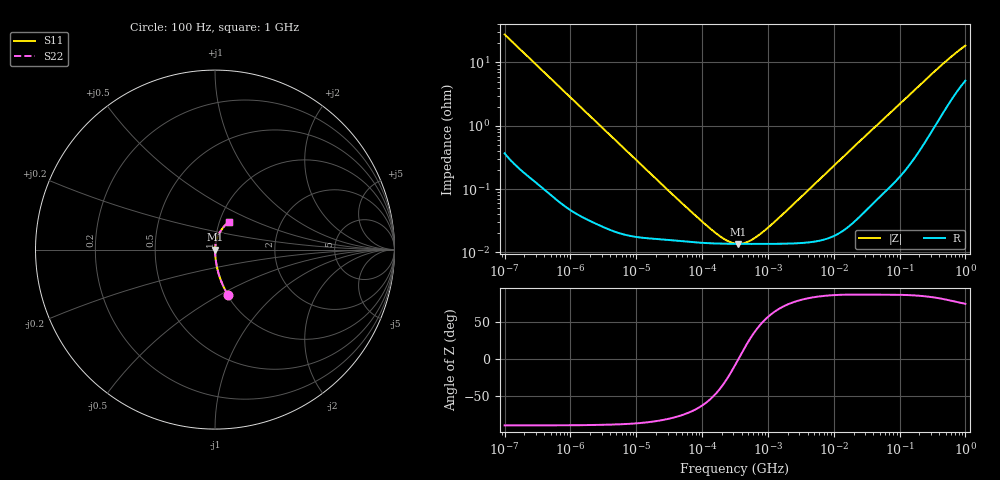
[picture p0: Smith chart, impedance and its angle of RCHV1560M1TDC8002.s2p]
! RCHV1560M1TDC8002  S-PARAMETER MODEL  (AEC-Q200 qualified)
! Model Generated by ELNA Corporation (http://www.ty-top.com)
! Version 1.0
! ELNA Control No. 240229
! Copyright (c) 2024 ELNA CO.,LTD. All Rights Reserved.
! Products Name : CONDUCTIVE POLYMER HYBRID ALUMINUM ELECTROLYTIC CAPACITORS
! Characteristics :
!  Capacitance  :  56uF  ,  Rated voltage  :  25V
!  Operating Temp. Range  :  -55 to +105 degC  ,  Endurance  :  5000hr at 105 degC
!  Dimension D  :  6.3mm  ,  Dimension L  :  5.8mm
! Frequency Range : 100Hz - 1GHz
! External Node Assignments :
!  1  o---| |---o  2
# MHz S RI R 50
!Freq[MHz].  S11 Real  S11 Imag  S21 Real  S21 Imag  S12 Real  S12 Imag  S22 Real  S22 Imag
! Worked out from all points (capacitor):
!   401 points, 100 Hz to 1 GHz, reference 50 ohm
!   read as one part in series: C = 57.5 uF near 108 Hz
!   lowest |Z| = 13.6 mohm at 356.9 kHz (marker M1)
!   series resonance near 357.6 kHz, so ESL is about 3.4 nH
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0.0001  0.074 -0.2553  0.926 0.2553  0.926 0.2553  0.074 -0.2553
0.000113  0.0594 -0.23  0.9406 0.23  0.9406 0.23  0.0594 -0.23
0.000183  0.0242 -0.1476  0.9758 0.1476  0.9758 0.1476  0.0242 -0.1476
0.000309  0.00924 -0.0891  0.9908 0.0891  0.9908 0.0891  0.00924 -0.0891
0.000613  0.00275 -0.0455  0.9972 0.0455  0.9972 0.0455  0.00275 -0.0455
0.001488  0.000722 -0.0189  0.9993 0.0189  0.9993 0.0189  0.000722 -0.0189
0.022131  0.000163 -0.00129  0.9998 0.00129  0.9998 0.00129  0.000163 -0.00129
0.074131  0.000145 -0.00038  0.9999 0.00038  0.9999 0.00038  0.000145 -0.00038
0.147062  0.000139 -0.000168  0.9999 0.000168  0.9999 0.000168  0.000139 -0.000168
0.229087  0.000137 -7.67e-05  0.9999 7.67e-05  0.9999 7.67e-05  0.000137 -7.67e-05
0.316228  0.000136 -2.06e-05  0.9999 2.06e-05  0.9999 2.06e-05  0.000136 -2.06e-05
0.356862  0.000136 -3.51e-07  0.9999 3.51e-07  0.9999 3.51e-07  0.000136 -3.51e-07
0.419276  0.000136 2.67e-05  0.9999 -2.67e-05  0.9999 -2.67e-05  0.000136 2.67e-05
0.512861  0.000136 6.15e-05  0.9999 -6.15e-05  0.9999 -6.15e-05  0.000136 6.15e-05
0.767361  0.000136 0.00014  0.9999 -0.00014  0.9999 -0.00014  0.000136 0.00014
1.40443  0.000137 0.000307  0.9999 -0.000307  0.9999 -0.000307  0.000137 0.000307
4.704354  0.000147 0.00109  0.9999 -0.00109  0.9999 -0.00109  0.000147 0.00109
69.9842  0.00129 0.0154  0.9987 -0.0154  0.9987 -0.0154  0.00129 0.0154
184.0772  0.00506 0.0394  0.9949 -0.0394  0.9949 -0.0394  0.00506 0.0394
412.0975  0.0202 0.0826  0.9798 -0.0826  0.9798 -0.0826  0.0202 0.0826
695.825  0.0466 0.1244  0.9534 -0.1244  0.9534 -0.1244  0.0466 0.1244
1000  0.0753 0.1562  0.9247 -0.1562  0.9247 -0.1562  0.0753 0.1562
